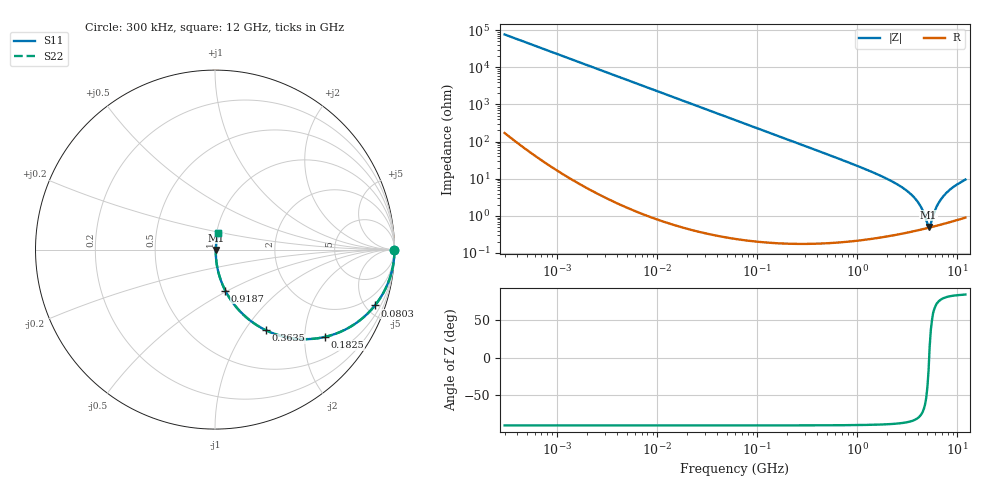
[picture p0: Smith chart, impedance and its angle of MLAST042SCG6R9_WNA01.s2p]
! MLAST042SCG6R9_WNA01  S-PARAMETER MODEL  ( General Type )
! Model Generated by TAIYO YUDEN Corporation (http://www.ty-top.com)
! Version 1.0
! TAIYO YUDEN Control No. 150820
! Copyright(c) 2015 TAIYO YUDEN CO.,LTD. All Rights Reserved.
! Product Description (link to TY-COMPAS)
! https://ds.yuden.co.jp/TYCOMPAS/or/detail?pn=MLAST042SCG6R9BWNA01&u=M
! Products Name : Multilayer Ceramic Capacitors
! Characteristics :
!  Capacitance : 6.9 pF , Rated Voltage : 25V , TCC : CG / C0G
!  Case Size : 0.4 x 0.2 / 0.016 x 0.008 [mm/inch] , Thickness : 0.2 / 0.008 [mm/inch]
!  (Conditions: Temperature = 25 degC , DC Bias Current/Voltage = 0A / 0V)
! External Node Assignments :
!  1  o---| |---o  2
! GND o---------o GND
! Frequency Range : 0.3MHz  -  12000MHz  [ 401 STEP ]
# MHz S RI R 50
! Freq[MHz].  S11 Real  S11 Imag  S21 Real  S21 Imag  S12 Real  S12 Imag  S22 Real  S22 Imag
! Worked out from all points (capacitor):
!   401 points, 300 kHz to 12 GHz, reference 50 ohm
!   read as one part in series: C = 6.92 pF near 316.3 kHz
!   lowest |Z| = 501 mohm at 5.141 GHz (marker M1)
!   series resonance near 5.214 GHz, so ESL is about 130 pH
!   S11 on the Smith chart (normalised r, x): 300 kHz: open; 80.3 MHz: 1.00, -5.73; 182.5 MHz: 1.00, -2.52; 363.5 MHz: 1.00, -1.26; 918.7 MHz: 1.00, -0.49; 12 GHz: 1.02, +0.19
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0.3  1 -0.0013  4.6e-06 0.0013  4.6e-06 0.0013  1 -0.0013
1.769972  0.9999 -0.0077  6.32e-05 0.0077  6.32e-05 0.0077  0.9999 -0.0077
10.44266  0.9979 -0.0453  0.00207 0.0453  0.00207 0.0453  0.9979 -0.0453
27.10171  0.9863 -0.1162  0.0137 0.1162  0.0137 0.1162  0.9863 -0.1162
60  0.9361 -0.2442  0.0639 0.2442  0.0639 0.2442  0.9361 -0.2442
80.29859  0.8911 -0.3111  0.1089 0.3111  0.1089 0.3111  0.8911 -0.3111
182.544  0.6128 -0.4864  0.3872 0.4864  0.3872 0.4864  0.6128 -0.4864
353.9943  0.2954 -0.4549  0.7046 0.4549  0.7046 0.4549  0.2954 -0.4549
363.4975  0.2845 -0.4497  0.7155 0.4497  0.7155 0.4497  0.2845 -0.4497
570.2811  0.1382 -0.3428  0.8618 0.3428  0.8618 0.3428  0.1382 -0.3428
918.7169  0.0573 -0.2282  0.9427 0.2282  0.9427 0.2282  0.0573 -0.2282
2088.533  0.0113 -0.0912  0.9887 0.0912  0.9887 0.0912  0.0113 -0.0912
2947.191  0.0062 -0.0527  0.9938 0.0527  0.9938 0.0527  0.0062 -0.0527
3740.715  0.00479 -0.0297  0.9952 0.0297  0.9952 0.0297  0.00479 -0.0297
4270.516  0.00454 -0.0178  0.9955 0.0178  0.9955 0.0178  0.00454 -0.0178
5006.236  0.00469 -0.00378  0.9953 0.00378  0.9953 0.00378  0.00469 -0.00378
5140.631  0.00476 -0.0015  0.9952 0.0015  0.9952 0.0015  0.00476 -0.0015
5420.343  0.00494 0.00375  0.9951 -0.00375  0.9951 -0.00375  0.00494 0.00375
6188.031  0.00568 0.0168  0.9943 -0.0168  0.9943 -0.0168  0.00568 0.0168
7254.098  0.00715 0.0333  0.9928 -0.0333  0.9928 -0.0333  0.00715 0.0333
8966.534  0.0104 0.0571  0.9896 -0.0571  0.9896 -0.0571  0.0104 0.0571
12000  0.0176 0.0922  0.9824 -0.0922  0.9824 -0.0922  0.0176 0.0922
